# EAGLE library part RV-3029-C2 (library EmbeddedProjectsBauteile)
Real Time Clock Module with I2C-Bus
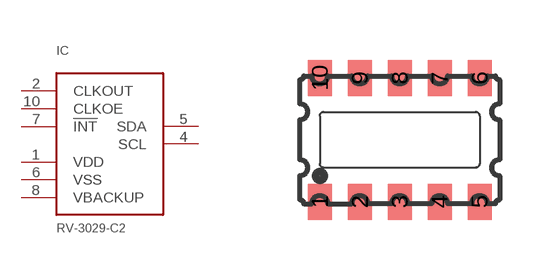
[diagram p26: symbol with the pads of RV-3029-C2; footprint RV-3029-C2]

Designator prefix IC

## RV-3029-C2 (EP: 400243)  [RV-3029-C2]
1  VDD
2  CLKOUT
4  SCL
5  SDA
6  VSS
7  !INT
8  VBACKUP
10  CLKOE

## Footprint RV-3029-C2 (pad centres in mm)
smd 0.6 x 0.9: 1 -2,-1.55; 2 -1,-1.55; 3 0,-1.55; 4 1,-1.55; 5 2,-1.55; 6 2,1.55; 7 1,1.55; 8 0,1.55; 9 -1,1.55; 10 -2,1.55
